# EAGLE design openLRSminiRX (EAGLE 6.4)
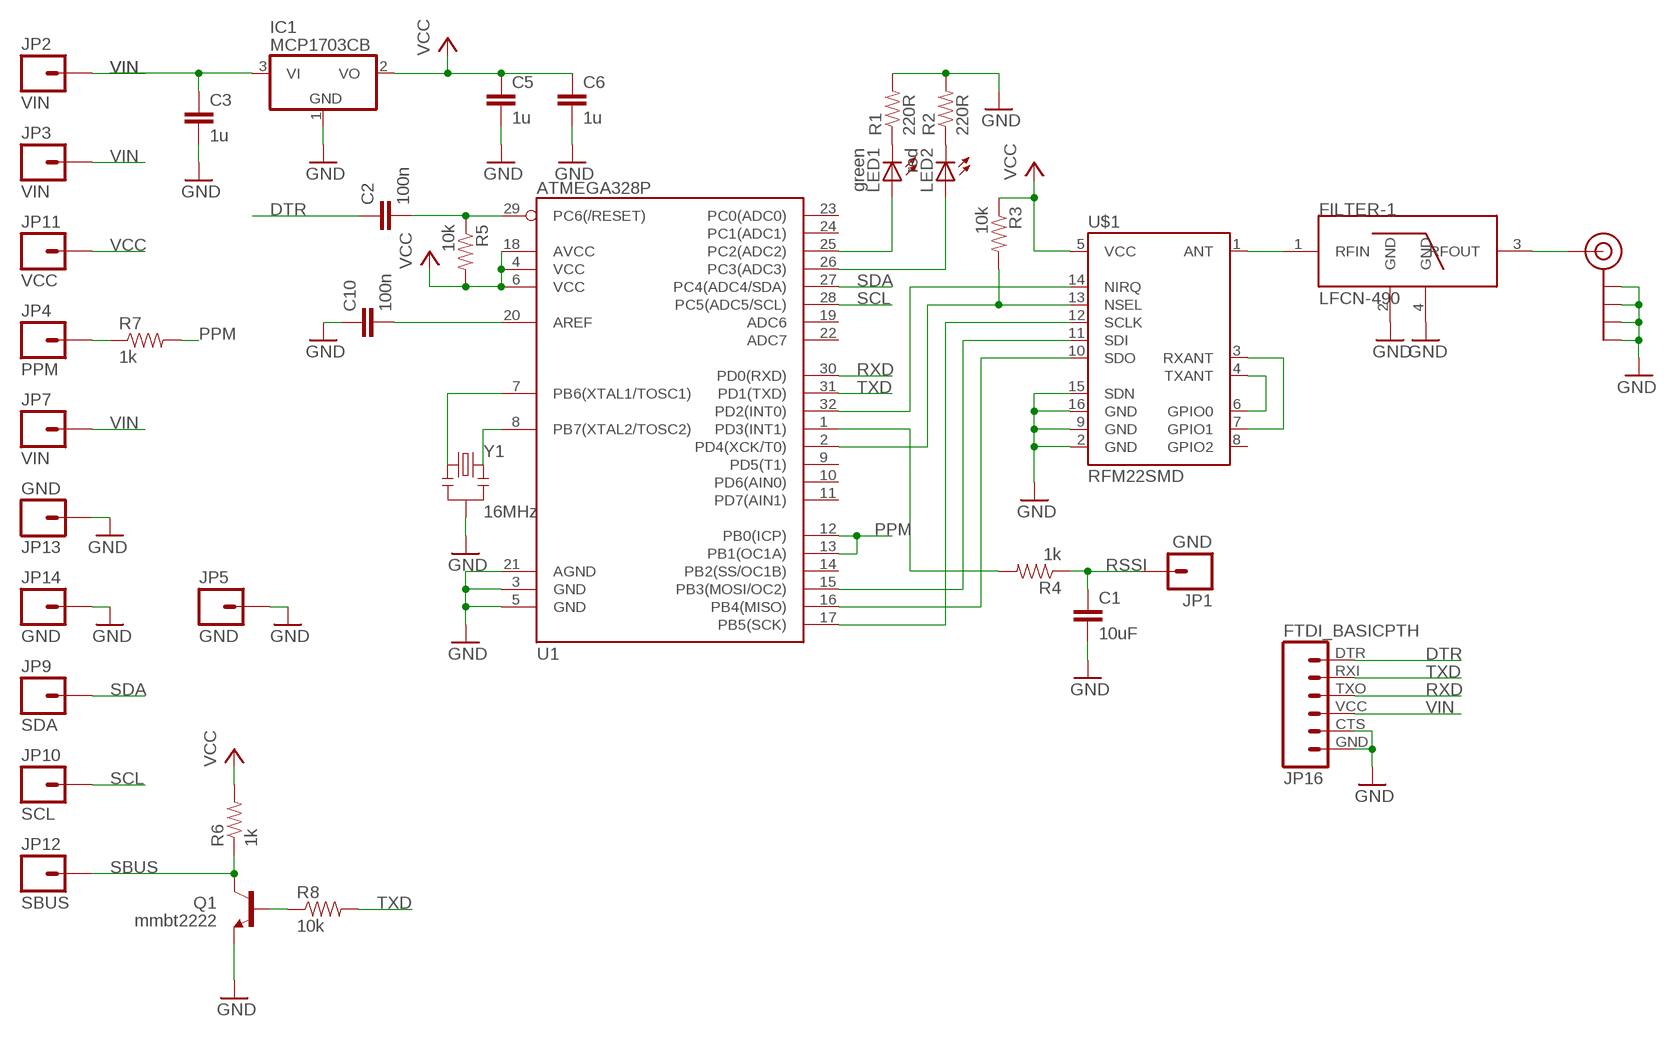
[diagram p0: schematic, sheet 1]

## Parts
C1  10uF  CAP0805  [0805]
C2  100n  CAP0805  [0805]
C3  1u  CAP0805  [0805]
C5  1u  CAP0805  [0805]
C6  1u  CAP0805  [0805]
C10  100n  CAP0805  [0805]
FILTER-1  LFCN-490  [FV1206]
IC1  MCP1703CB  [SOT23]
J$1  SMA_EDGE  [SMA-EDGE]
JP1  GND  M01PTH  [1X01]
JP2  VIN  M01PTH  [1X01]
JP3  VIN  M01PTH  [1X01]
JP4  PPM  M01PTH  [1X01]
JP5  GND  M01PTH  [1X01]
JP7  VIN  M01PTH  [1X01]
JP9  SDA  M01PTH  [1X01]
JP10  SCL  M01PTH  [1X01]
JP11  VCC  M01PTH  [1X01]
JP12  SBUS  M01PTH  [1X01]
JP13  GND  M01PTH  [1X01]
JP14  GND  M01PTH  [1X01]
JP16  FTDI_BASICPTH  [FTDI_BASIC]
LED1  green  LEDSML0805  [SML0805]
LED2  red  LEDSML0805  [SML0805]
Q1  mmbt2222  TRANSISTOR_NPNSOT23  [SOT23]
R1  220R  RESISTOR0805-RES  [0805]
R2  220R  RESISTOR0805-RES  [0805]
R3  10k  RESISTOR0805-RES  [0805]
R4  1k  RESISTOR0805-RES  [0805]
R5  10k  RESISTOR0805-RES  [0805]
R6  1k  RESISTOR0805-RES  [0805]
R7  1k  RESISTOR0805-RES  [0805]
R8  10k  RESISTOR0805-RES  [0805]
U1  ATMEGA328P  ATMEGA328_SMT  [TQFP32-08]
U$1  RFM22SMD  [RFM22-XXX-S2]
Y1  16MHz  RESONATOR16MHZ  [RESONATOR-SMD]

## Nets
DTR: C2.1 JP16.DTR
GND: C1.2 C3.2 C5.2 C6.2 C10.1 FILTER-1.2(GND) FILTER-1.4(GND) IC1.1(GND) J$1.GND@0(GND) J$1.GND@1(GND) J$1.GND@2(GND) J$1.GND@3(GND) JP5.1 JP13.1 JP14.1 JP16.CTS JP16.GND Q1.2(E) R1.2 R2.2 U1.3(GND) U1.5(GND) U1.21(AGND) U$1.2(GND) U$1.9(GND) U$1.15(SDN) U$1.16(GND) Y1.2
N$1: FILTER-1.1(RFIN) U$1.1(ANT)
N$2: U$1.4(TXANT) U$1.6(GPIO0)
N$3: U$1.3(RXANT) U$1.7(GPIO1)
N$4: FILTER-1.3(RFOUT) J$1.SIG(SIGNAL)
N$5: JP4.1 R7.1
N$6: R4.2 U1.1(PD3(INT1))
N$7: U1.15(PB3(MOSI/OC2)) U$1.11(SDI)
N$8: U1.16(PB4(MISO)) U$1.10(SDO)
N$9: U1.17(PB5(SCK)) U$1.12(SCLK)
N$10: R3.2 U1.2(PD4(XCK/T0)) U$1.13(NSEL)
N$11: U1.32(PD2(INT0)) U$1.14(NIRQ)
N$12: LED1.C R1.1
N$13: LED2.C R2.1
N$14: LED1.A U1.25(PC2(ADC2))
N$15: LED2.A U1.26(PC3(ADC3))
N$16: U1.7(PB6(XTAL1/TOSC1)) Y1.1
N$17: U1.8(PB7(XTAL2/TOSC2)) Y1.3
N$18: C2.2 R5.1 U1.29(PC6(/RESET))
N$19: C10.2 U1.20(AREF)
N$21: Q1.1(B) R8.1
PPM: R7.2 U1.12(PB0(ICP)) U1.13(PB1(OC1A))
RSSI: C1.1 JP1.1 R4.1
RXD: JP16.TXO U1.30(PD0(RXD))
SBUS: JP12.1 Q1.3(C) R6.1
SCL: JP10.1 U1.28(PC5(ADC5/SCL))
SDA: JP9.1 U1.27(PC4(ADC4/SDA))
TXD: JP16.RXI R8.2 U1.31(PD1(TXD))
VCC: C5.1 C6.1 IC1.2(VO) JP11.1 R3.1 R5.2 R6.2 U1.4(VCC) U1.6(VCC) U1.18(AVCC) U$1.5(VCC)
VIN: C3.1 IC1.3(VI) JP2.1 JP3.1 JP7.1 JP16.VCC
Unconnected: U1.9(PD5(T1)) U1.10(PD6(AIN0)) U1.11(PD7(AIN1)) U1.14(PB2(SS/OC1B)) U1.19(ADC6) U1.22(ADC7) U1.23(PC0(ADC0)) U1.24(PC1(ADC1)) U$1.8(GPIO2)

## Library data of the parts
C1-C3 C5 C6 C10 = SparkFun-Capacitors:CAP: Capacitor
FILTER-1 = minicircuits:LFCN: Low pass Filter Features: Excellent power handling: 8/9 W (depending on reference) Max DC current 0.5A/1A (depending on reference) Small size 5/7 sections (depending on reference) Operating temperature: -55°C - 100°C Applications: Harmonic rejection VHF/UHF transmitters/receivers Lab use
IC1 = linear:MCP1703: 250 mA, 16V, Low Quiescent Current LDO Regulator Source: http://ww1.microchip.com/downloads/en/DeviceDoc/22049b.pdf
J$1 = SparkFun:SMA_EDGE: SMA Antenna Connector End launch SMA connector. The paste layer has been removed so that the connector can be hand soldered onto the board after reflow.
JP1-JP5 JP7 JP9-JP14 = SparkFun-Connectors:M01: Header 1
JP16 = SparkFun:FTDI_BASIC: FTDI Basic: 3.3V and 5V
LED1 LED2 = led:LED: LED
Q1 = SparkFun-DiscreteSemi:TRANSISTOR_NPN: Generic NPN BJT. MMBT2222 is the common NPN we use. Double check against datasheet- not all devices are the same!
R1-R8 = SparkFun-Resistors:RESISTOR: Resistor
U1 = SparkFun-DigitalIC:ATMEGA328_SMT: 32-Pin Atmega328 part Commonly used on Arduino compatible boards Available in QFP and QFN packages TQFP is IC-09069 QFN is non-stock; PROD_ID: IC-09069
U$1 = SparkFun-RF:RFM22: The RFM22 is a low-power, low cost radio that is capable of operating in the 434MHz and 900MHz open bands. It's frequency is software defined and there are some very good libraries written for it.
Y1 = SparkFun-FreqCtrl:RESONATOR: Resonator Small SMD resonator. Used, eg, on the Arduino Pro/ Pro Mini boards. 8MHz- XTAL-08895 16MHz- XTAL-08900; PROD_ID: XTAL-08900

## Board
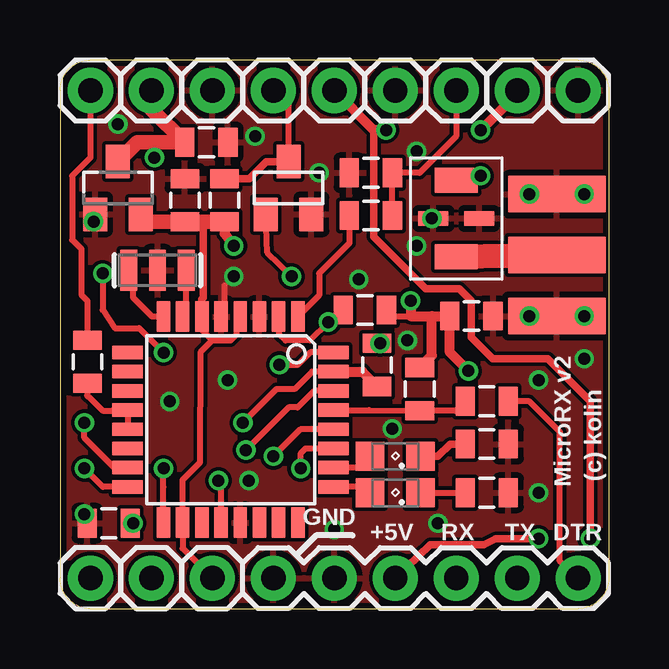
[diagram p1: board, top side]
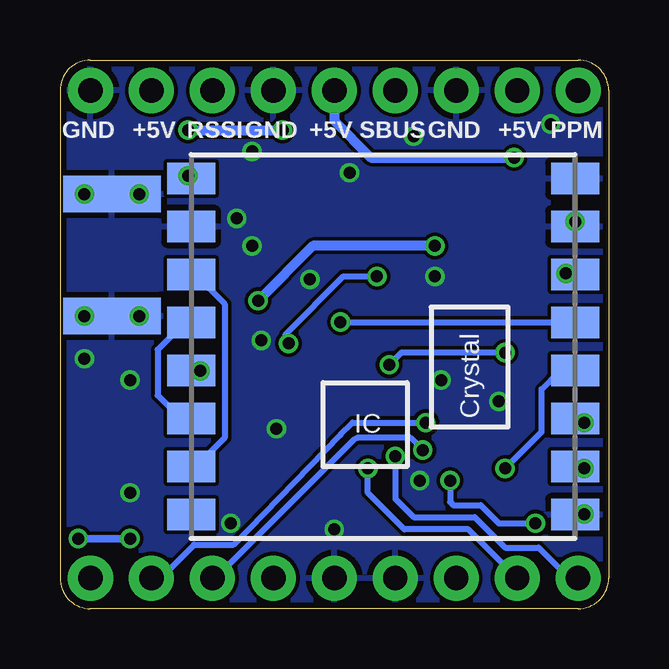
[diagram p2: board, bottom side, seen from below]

Size 22.86 x 22.86 mm. Coordinates in mm from the lower left corner, seen from the top.
Outline: 1.27,0 21.59,0 arc90 22.86,1.27 22.86,21.59 arc90 21.59,22.86 1.27,22.86 arc90 0,21.59 0,1.27 arc90 1.27,0
Copper layers (1*16): Top 0.035mm / dielectric 1.5mm / Bottom 0.035mm
Design rules "ITEADstudio_DRC": minimum track width 6mil, minimum drill 12mil, track to track 6mil, track to pad 6mil, pad to pad 6mil, via to via 6mil, smd to smd 0mil, copper to edge 10mil, drill to drill 10mil, minimum pad ring 10mil, minimum via ring 6mil, stop-mask expansion 2mil, vias tented up to drill 100mil, thermal gap 10mil

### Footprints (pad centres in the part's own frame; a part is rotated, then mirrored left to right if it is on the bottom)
0805 = smd 0.8 x 1.2: 1 -0.9,0; 2 0.9,0
FV1206 = smd 1.041 x 1.803: 1 -1.587,0; 3 1.587,0 | smd 0.61 x 1.245: 2 0,-0.953; 4 0,0.953
SOT23 = smd 1 x 1.4: 1 -0.95,-1.1; 2 0.95,-1.1; 3 0,1.1
SMA-EDGE = smd 1.524 x 4.064: GND@0 0,0; GND@1 5.08,0; SIG 2.54,0 | smd 1.524 x 4.064 bottom: GND@2 0,0; GND@3 5.08,0
1X01 = drill 1.016 pad 1.88: 1 0,0
FTDI_BASIC = drill 1.016 pad 1.88: CTS 10.16,0; DTR 0,0; GND 12.7,0; RXI 2.54,0; TXO 5.08,0; VCC 7.62,0
SML0805 = smd 1.2 x 1.2: A 1.05,0; C -1.05,0
TQFP32-08 = smd 1.27 x 0.559: 1 -4.293,2.8; 2 -4.293,2; 3 -4.293,1.2; 4 -4.293,0.4; 5 -4.293,-0.4; 6 -4.293,-1.2; 7 -4.293,-2; 8 -4.293,-2.8; 17 4.293,-2.8; 18 4.293,-2; 19 4.293,-1.2; 20 4.293,-0.4; 21 4.293,0.4; 22 4.293,1.2; 23 4.293,2; 24 4.293,2.8 | smd 0.559 x 1.27: 9 -2.8,-4.293; 10 -2,-4.293; 11 -1.2,-4.293; 12 -0.4,-4.293; 13 0.4,-4.293; 14 1.2,-4.293; 15 2,-4.293; 16 2.8,-4.293; 25 2.8,4.293; 26 2,4.293; 27 1.2,4.293; 28 0.4,4.293; 29 -0.4,4.293; 30 -1.2,4.293; 31 -2,4.293; 32 -2.8,4.293
RFM22-XXX-S2 = smd 2 x 1.3: 1 -8,7; 2 -8,5; 3 -8,3; 4 -8,1; 5 -8,-1; 6 -8,-3; 7 -8,-5; 8 -8,-7; 9 8,-7; 10 8,-5; 11 8,-3; 12 8,-1; 13 8,1; 14 8,3; 15 8,5; 16 8,7
RESONATOR-SMD = smd 0.7 x 1.7: 1 -1.2,0; 2 0,0; 3 1.2,0

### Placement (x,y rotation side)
C1  12.95,18.16 180 top
C2  17.78,8.64 180 top
C3  6.1,19.43 0 top
C5  17.14,12.19 0 top
C6  5.21,17.02 90 top
C10  2.03,3.56 0 top
FILTER-1  16.51,16.26 270 top
IC1  2.41,17.53 0 top
J$1  20.7,12.19 90 top
JP1  16.51,21.59 0 top
JP2  19.05,21.59 0 top
JP3  11.43,21.59 0 top
JP4  1.27,21.59 0 top
JP5  13.97,21.59 0 top
JP7  3.81,21.59 0 top
JP9  3.81,1.27 0 top
JP10  1.27,1.27 0 top
JP11  6.35,1.27 0 top
JP12  8.89,21.59 0 top
JP13  21.59,21.59 0 top
JP14  6.35,21.59 0 top
JP16  21.59,1.27 180 top
LED1  13.97,4.83 180 top
LED2  13.97,6.35 180 top
Q1  9.53,17.53 0 top
R1  17.78,4.83 0 top
R2  17.78,6.86 0 top
R3  12.7,12.45 180 top
R4  12.95,16.38 180 top
R5  14.99,9.14 90 top
R6  6.86,17.02 270 top
R7  1.14,10.29 270 top
R8  13.21,10.16 270 top
U1  7.11,7.87 270 top
U$1  9.4,10.92 0 bottom
Y1  4.06,14.1 180 top

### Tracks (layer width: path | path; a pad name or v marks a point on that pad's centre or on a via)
DTR
  Top 0.254: C2.1 19.56,8.64 20.83,7.37 20.83,1.97 JP16.DTR
GND  (via drill 0.5)
  Top 0.254: U1.5 6.86,12.17 6.86,13.46
  other vias: 19.94,4.83 11.43,3.3 14.48,11.18 8.13,19.68 10.79,18.16 7.24,13.84 15.49,16.26 6.99,9.53 12.45,13.72 7.87,5.33 2.41,20.19 4.57,8.64 1.02,3.94 14.86,19.05 1.4,16.13 19.94,9.53 21.84,10.41 19.56,12.19 21.84,12.19 19.56,17.27 21.84,17.27 14.86,15.11 13.84,7.49 15.75,3.56
  pour Bottom: 0,0 22.86,0 22.86,22.86 0,22.86
  pour Top: 0,0 22.86,0 22.86,22.86 0,22.86
N$1  (via drill 0.5 pad 0.25)
  Top 0.406: v17.53,18.03 FILTER-1.1
  Bottom 0.406: U$1.1 v17.53,18.03
N$2
  Bottom 0.254: U$1.4 17.8,11.79 18.8,10.79 18.8,8.89 18.29,8.38 17.86,8.38 U$1.6
N$3
  Bottom 0.254: U$1.3 17.22,13.92 16,12.7 16,7.11 16.76,6.35 16.97,6.35 U$1.7
N$4
  Top 1.016: FILTER-1.3 19.88,14.73 J$1.SIG
N$5
  Top 0.254: JP4.1 1.27,18.8 0.51,18.03 0.51,15.37 0.89,14.99 0.89,13.08 1.14,12.83 R7.1
N$6
  Top 0.254: R4.2 12.05,15.23 10.79,13.97 10.79,13.05 U1.1
N$7  (via drill 0.5)
  Top 0.254: U1.15 2.25,5.87 1.02,7.11 v1.02,7.75
  Bottom 0.254: v1.02,7.75 1.1,7.62 U$1.11
N$8  (via drill 0.5)
  Top 0.254: U1.16 1.78,5.07 v1.02,5.84
  Bottom 0.254: v1.02,5.84 1.06,5.59 U$1.10
N$9  (via drill 0.5)
  Top 0.254: U1.17 4.31,5.07 v4.32,5.84
  Bottom 0.254: v4.32,5.84 2.79,7.37 2.79,9.14 2.03,9.91 1.41,9.91 U$1.12
N$10  (via drill 0.5)
  Top 0.254: v11.18,11.94 11.68,12.45 R3.2 11.24,11.94 v11.18,11.94 | v11.18,11.94 10.41,11.18 9.4,11.18 9.14,11.43 9.14,12.13 U1.2
  Bottom 0.254: U$1.13 11.16,11.92 v11.18,11.94
N$11  (via drill 0.5)
  Top 0.254: U1.32 10.42,10.67 9.91,10.16 v9.14,10.16 | v1.78,13.97 1.78,12.45 2.29,11.68 3.3,11.68 v4.32,10.67
  Bottom 0.254: v4.32,10.67 8.64,10.67 v9.14,10.16 | v1.78,13.97 1.45,13.97 U$1.14
N$12
  Top 0.254: LED1.C R1.1
N$13
  Top 0.305: LED2.C 15.75,6.35 16.26,6.86 R2.1
N$14
  Top 0.254: LED1.A 12.67,5.07 U1.25
N$15
  Top 0.254: LED2.A 12.44,5.87 U1.26
N$16
  Top 0.254: U1.7 5.26,12.17 Y1.1
N$17
  Top 0.254: U1.8 3.83,12.17 3.05,12.95 3.05,13.79 Y1.3
N$18
  Top 0.254: U1.29 12.87,8.27 R5.1 16.49,8.24 C2.2
N$19  (via drill 0.5)
  Top 0.254: U1.20 6.71,5.23 v6.6,5.33 | v3.05,3.56 C10.2
  Bottom 0.254: v6.6,5.33 6.6,4.45 6.48,4.32 5.33,4.32 4.57,3.56 v3.05,3.56
N$21  (via drill 0.5)
  Top 0.254: R8.1 v13.35,11.06 v13.34,11.05 | v9.65,13.84 8.64,14.84 Q1.1
  Bottom 0.254: v13.34,11.05 13.46,11.43 11.05,13.84 v9.65,13.84
PPM
  Top 0.254: R7.2 1.13,8.88 1.27,8.76 1.78,8.26 2.17,8.26 U1.12 U1.13
RSSI
  Top 0.254: R4.1 C1.1 | C1.1 13.97,18.28 | JP1.1 16.51,19.68 14.99,18.16 C1.1
RXD  (via drill 0.5)
  Top 0.254: U1.30 10.6,9.07 9.91,8.38 9.53,8.38 v7.75,6.6
  Bottom 0.254: v7.75,6.6 8.26,7.11 10.48,7.11 10.6,7.05 16.38,1.27 JP16.TXO
SBUS
  Top 0.254: Q1.3 9.53,20.95 JP12.1
  Top 0.305: R6.1 7.88,17.92 8.59,18.63 Q1.3
SCL  (via drill 0.5)
  Top 0.254: U1.28 10.01,7.47 v8.89,6.35
  Bottom 0.254: v8.89,6.35 8.89,4.57 8.13,3.81 5.59,3.81 4.32,2.54 2.92,2.54 1.65,1.27 JP10.1
SDA  (via drill 0.5)
  Top 0.254: v10.03,5.84 10.03,6.48 10.23,6.67 U1.27
  Bottom 0.254: JP9.1 5.84,3.3 8.51,3.3 10.03,4.83 v10.03,5.84
TXD  (via drill 0.5)
  Top 0.254: U1.31 10.51,9.87 9.78,9.14 9.02,9.14 v7.62,7.75
  Top 0.406: U1.31 12.59,9.87 R8.2
  Bottom 0.254: JP16.RXI 18.61,1.33 17.27,2.67 15.62,2.67 11.18,7.24 10.67,7.75 v7.62,7.75
VCC  (via drill 0.5)
  Top 0.254: U1.6 5.91,11.61 6.35,11.18 | 6.35,11.18 7.11,11.18 7.37,11.43 7.37,12.02 U1.4 | 6.35,11.18 5.87,10.7 5.84,6.1 5.11,5.37 U1.18 5.11,2.51 JP11.1 | R3.1 13.59,12.19 14.61,12.19
  Top 0.305: U1.6 5.91,12.9 5.97,12.95 5.97,15.99 6.1,16.12
  Top 0.406: v14.61,12.83 14.61,12.19 15.49,12.19 | 15.49,12.19 C5.1 16.25,10.68 v17.02,9.91 | R5.2 15.49,10.55 15.49,12.19 | R6.2 6.86,15.62 v7.24,15.11
  Top 0.61: IC1.2 3.67,16.12 C6.1 6.1,16.12 R6.2
  Bottom 0.406: v7.24,15.11 12.32,15.11 v14.61,12.83 | 17.78,9.91 17.76,9.92 U$1.5 17.53,10.05 v17.02,9.91
VIN  (via drill 0.5)
  Top 0.305: 13.08,19.94 13.08,15.49 15.24,13.34 16.64,13.34 17.14,12.83 17.14,11.3 18.03,10.41 20.32,10.41 22.1,8.64 v22.1,2.92 | v19.94,2.92 18.16,2.92 17.65,2.67 15.43,2.67 JP16.VCC
  Top 0.406: JP2.1 19.05,21.46 v17.53,19.94 | v13.59,19.94 13.08,19.94 JP3.1 | v3.94,18.8 3.94,19.43
  Top 0.61: JP7.1 3.81,20.82 C3.1 3.94,19.43 3.22,19.43 IC1.3
  Bottom 0.305: v22.1,2.92 v19.94,2.92
  Bottom 0.406: v17.53,19.94 v13.59,19.94 | JP3.1 11.43,20.32 9.91,18.8 v3.94,18.8

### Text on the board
tPlace: MicroRX v2 | (c) kolin | GND | +5V | RX | TX | DTR
bPlace: PPM | +5V | GND | SBUS | +5V | GND | RSSI | +5V | GND
tDocu: PPM | +5V | GND | SBUS | +5V | GND | RSSI | +5V | GND | SCL | SDA | 3V3 | GND | CTS | +5V | RX | TX | DTR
